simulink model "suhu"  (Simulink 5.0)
settings: Solver=ode45  StartTime=0.0  StopTime=400.0  RelTol=1e-3

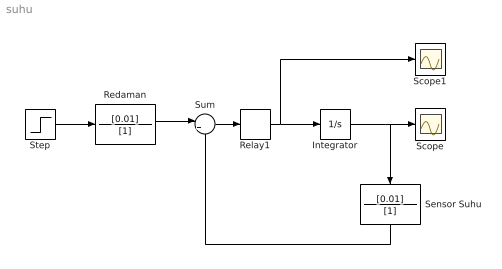
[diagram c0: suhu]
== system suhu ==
  Integrator : Integrator  InitialCondition=30
  Redaman : TransferFcn  Numerator=[0.01]  Denominator=[1]
  Relay1 : Relay  OnSwitchValue=0.02  OffSwitchValue=-0.02  OnOutputValue=0.5  OffOutputValue=-0.05
  Scope : Scope
  Scope1 : Scope
  Sensor Suhu : TransferFcn  Orientation=down  Numerator=[0.01]  Denominator=[1]
  Step : Step  After=40  SampleTime=0
  Sum : Sum  Inputs=|+-
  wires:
  Sum/1 -> Relay1/1
  Relay1/1 -> Scope1/1, Integrator/1
  Sensor Suhu/1 -> Sum/2
  Integrator/1 -> Scope/1, Sensor Suhu/1
  Step/1 -> Redaman/1
  Redaman/1 -> Sum/1
